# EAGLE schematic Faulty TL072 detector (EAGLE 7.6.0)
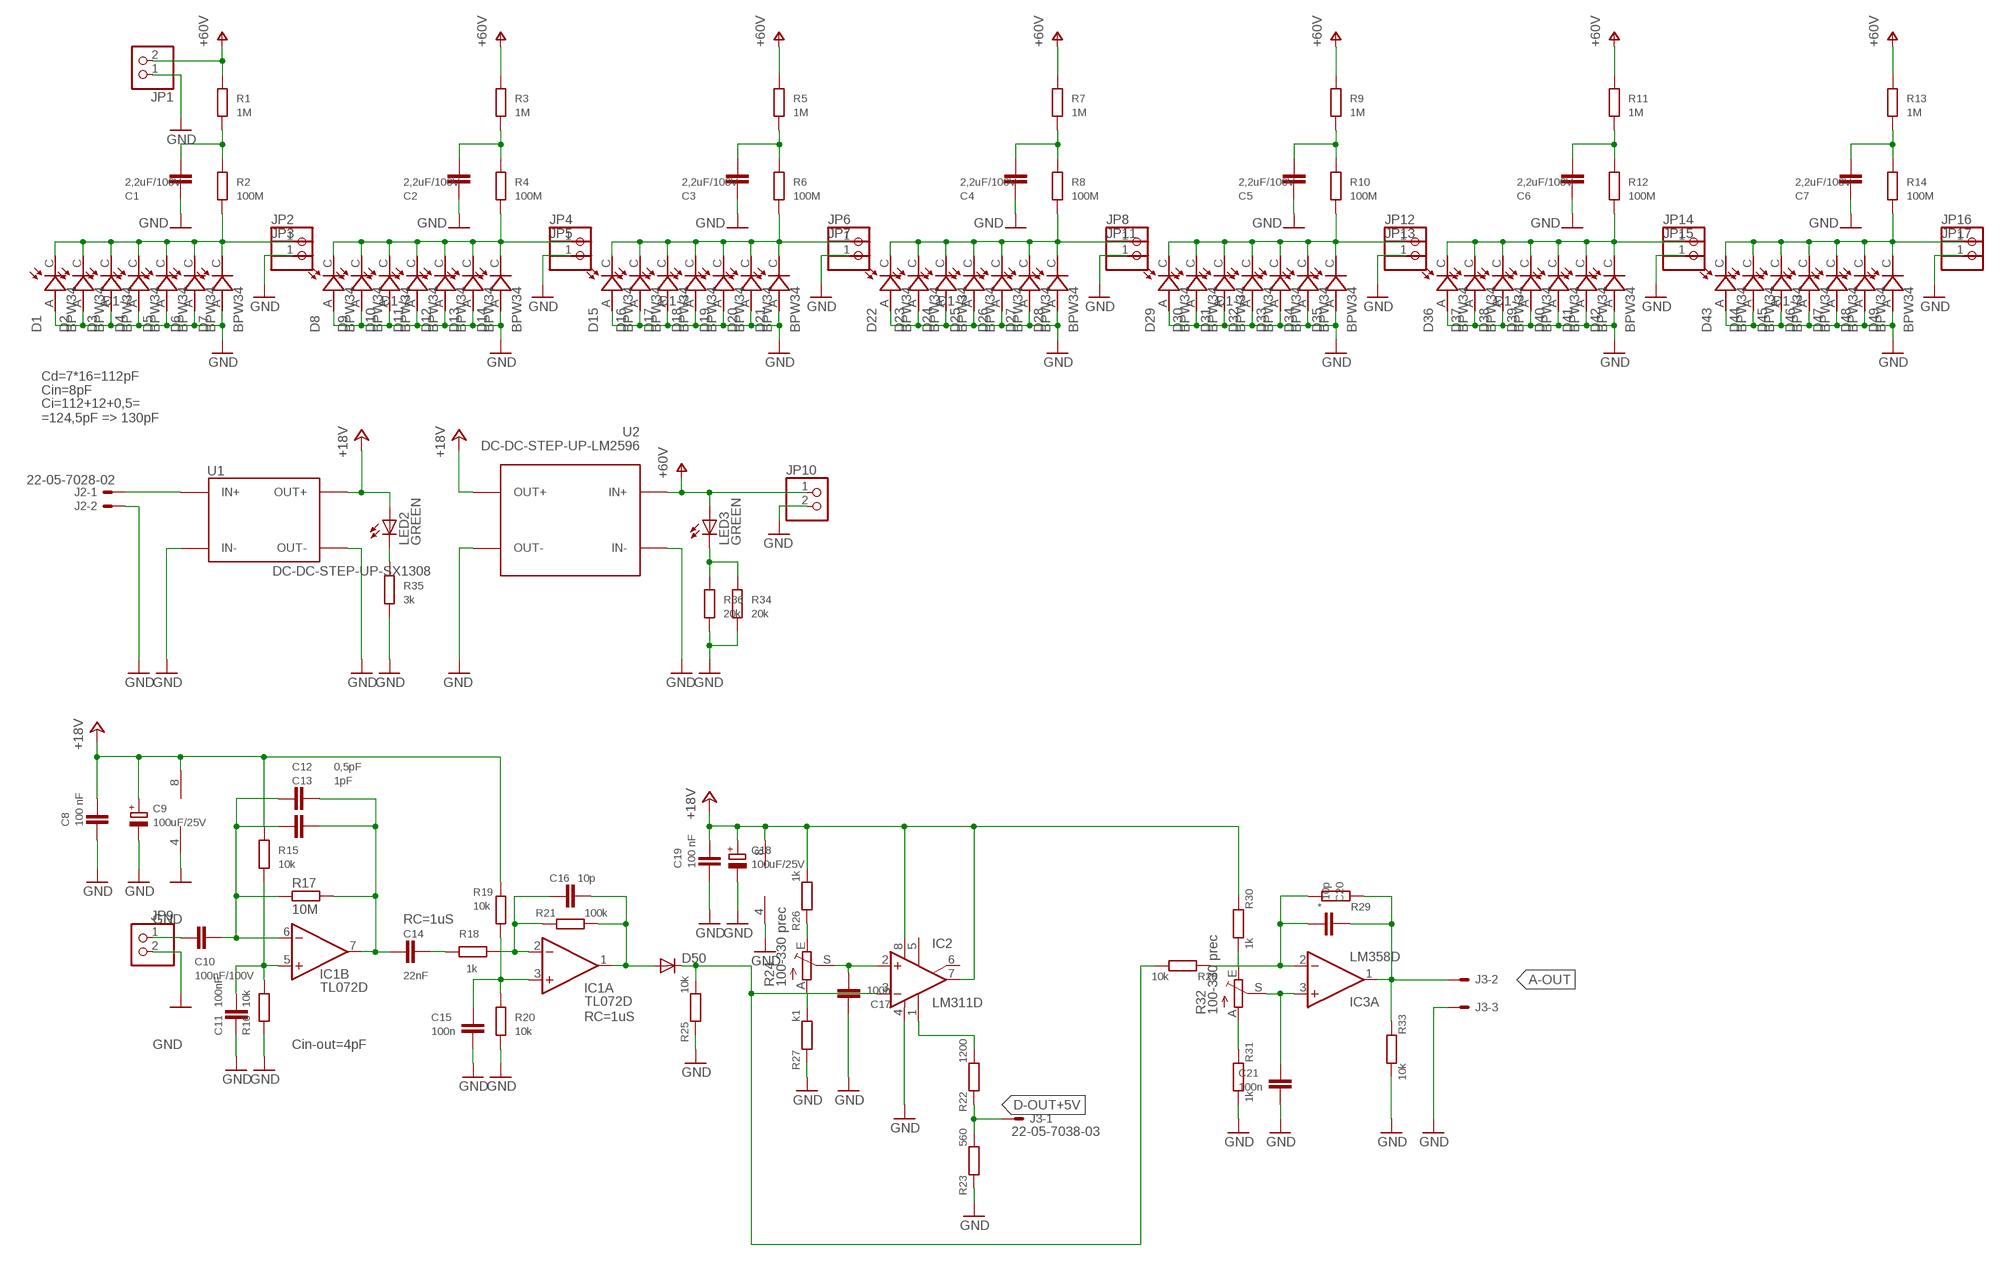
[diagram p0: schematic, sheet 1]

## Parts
C1  2,2uF/100V  C2824  [2824]
C2  2,2uF/100V  C2824  [2824]
C3  2,2uF/100V  C2824  [2824]
C4  2,2uF/100V  C2824  [2824]
C5  2,2uF/100V  C2824  [2824]
C6  2,2uF/100V  C2824  [2824]
C7  2,2uF/100V  C2824  [2824]
C8  100 nF  C-EUC0805  [C0805]
C9  100uF/25V  CPOL-EUSMCD  [SMC_D]
C10  100nF/100V  C-EUC1206  [C1206]
C11  100nF  C-EUC0805  [C0805]
C12  0,5pF  C-EUC0603  [C0603]
C13  1pF  C-EUC0805  [C0805]
C14  22nF  C-EUC0805  [C0805]
C15  100n  C-EUC0805  [C0805]
C16  10p  C-EUC0805  [C0805]
C17  100n  C-EUC0805  [C0805]
C18  100uF/25V  CPOL-EUSMCD  [SMC_D]
C19  100 nF  C-EUC0805  [C0805]
C20  10p  C-EUC0805  [C0805]
C21  100n  C-EUC0805  [C0805]
D1  BPW34  [PHODET_BPW34]
D2  BPW34  [PHODET_BPW34]
D3  BPW34  [PHODET_BPW34]
D4  BPW34  [PHODET_BPW34]
D5  BPW34  [PHODET_BPW34]
D6  BPW34  [PHODET_BPW34]
D7  BPW34  [PHODET_BPW34]
D8  BPW34  [PHODET_BPW34]
D9  BPW34  [PHODET_BPW34]
D10  BPW34  [PHODET_BPW34]
D11  BPW34  [PHODET_BPW34]
D12  BPW34  [PHODET_BPW34]
D13  BPW34  [PHODET_BPW34]
D14  BPW34  [PHODET_BPW34]
D15  BPW34  [PHODET_BPW34]
D16  BPW34  [PHODET_BPW34]
D17  BPW34  [PHODET_BPW34]
D18  BPW34  [PHODET_BPW34]
D19  BPW34  [PHODET_BPW34]
D20  BPW34  [PHODET_BPW34]
D21  BPW34  [PHODET_BPW34]
D22  BPW34  [PHODET_BPW34]
D23  BPW34  [PHODET_BPW34]
D24  BPW34  [PHODET_BPW34]
D25  BPW34  [PHODET_BPW34]
D26  BPW34  [PHODET_BPW34]
D27  BPW34  [PHODET_BPW34]
D28  BPW34  [PHODET_BPW34]
D29  BPW34  [PHODET_BPW34]
D30  BPW34  [PHODET_BPW34]
D31  BPW34  [PHODET_BPW34]
D32  BPW34  [PHODET_BPW34]
D33  BPW34  [PHODET_BPW34]
D34  BPW34  [PHODET_BPW34]
D35  BPW34  [PHODET_BPW34]
D36  BPW34  [PHODET_BPW34]
D37  BPW34  [PHODET_BPW34]
D38  BPW34  [PHODET_BPW34]
D39  BPW34  [PHODET_BPW34]
D40  BPW34  [PHODET_BPW34]
D41  BPW34  [PHODET_BPW34]
D42  BPW34  [PHODET_BPW34]
D43  BPW34  [PHODET_BPW34]
D44  BPW34  [PHODET_BPW34]
D45  BPW34  [PHODET_BPW34]
D46  BPW34  [PHODET_BPW34]
D47  BPW34  [PHODET_BPW34]
D48  BPW34  [PHODET_BPW34]
D49  BPW34  [PHODET_BPW34]
D50  DIODE-SOD323-W  [SOD323-W]
IC1  TL072D  [SO08]
IC2  LM311D  [SO08]
IC3  LM358D  [SO08]
J2  22-05-7028-02  [7395-02]
J3  22-05-7038-03  [7395-03]
JP1  PINHD-1X2  [1X02]
JP2  PINHD-1X1  [1X01]
JP3  PINHD-1X1  [1X01]
JP4  PINHD-1X1  [1X01]
JP5  PINHD-1X1  [1X01]
JP6  PINHD-1X1  [1X01]
JP7  PINHD-1X1  [1X01]
JP8  PINHD-1X1  [1X01]
JP9  PINHD-1X2  [1X02]
JP10  PINHD-1X2  [1X02]
JP11  PINHD-1X1  [1X01]
JP12  PINHD-1X1  [1X01]
JP13  PINHD-1X1  [1X01]
JP14  PINHD-1X1  [1X01]
JP15  PINHD-1X1  [1X01]
JP16  PINHD-1X1  [1X01]
JP17  PINHD-1X1  [1X01]
LED2  GREEN  LEDCHIPLED_1206  [CHIPLED_1206]
LED3  GREEN  LEDCHIPLED_1206  [CHIPLED_1206]
R1  1M  R-EU_M0805  [M0805]
R2  100M  R-EU_R0805  [R0805]
R3  1M  R-EU_M0805  [M0805]
R4  100M  R-EU_R0805  [R0805]
R5  1M  R-EU_M0805  [M0805]
R6  100M  R-EU_R0805  [R0805]
R7  1M  R-EU_M0805  [M0805]
R8  100M  R-EU_R0805  [R0805]
R9  1M  R-EU_M0805  [M0805]
R10  100M  R-EU_R0805  [R0805]
R11  1M  R-EU_M0805  [M0805]
R12  100M  R-EU_R0805  [R0805]
R13  1M  R-EU_M0805  [M0805]
R14  100M  R-EU_R0805  [R0805]
R15  10k  R-EU_R0805  [R0805]
R16  10k  R-EU_R0805  [R0805]
R17  10M  R-EU_R0805  [R0805]
R18  1k  R-EU_R0805  [R0805]
R19  10k  R-EU_R0805  [R0805]
R20  10k  R-EU_R0805  [R0805]
R21  100k  R-EU_R0805  [R0805]
R22  1200  R-EU_R0805  [R0805]
R23  560  R-EU_R0805  [R0805]
R24  100-330 prec  TRIM_EU-SP19L  [SP19L]
R25  10k  R-EU_R0805  [R0805]
R26  1k  R-EU_R0805  [R0805]
R27  k1  R-EU_R0805  [R0805]
R28  10k  R-EU_R0805  [R0805]
R29  *  R-EU_R0805  [R0805]
R30  1k  R-EU_R0805  [R0805]
R31  1k  R-EU_R0805  [R0805]
R32  100-330 prec  TRIM_EU-SP19L  [SP19L]
R33  10k  R-EU_R0805  [R0805]
R34  20k  R-EU_R0805  [R0805]
R35  3k  R-EU_R0805  [R0805]
R36  20k  R-EU_R0805  [R0805]
U1  DC-DC-STEP-UP-SX1308  [DC-DC-STEP-UP-SX1308]
U2  DC-DC-STEP-UP-LM2596  DC-DC-STEP-DOWN-LM2596  [DC-DC-STEP-DOWN-LM2596]

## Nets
+18V: C8.1 C9.+ C18.+ C19.1 IC1.8(P:V+) IC2.7(OUT) IC2.8(V+) IC3.8(P:V+) LED2.A R15.1 R19.1 R26.1 R30.2 U1.OUT+
+24V: U2.OUT+ ; supply symbol labelled +18V
+60: JP1.2 R1.1 R3.1 R5.1 R7.1 R9.1 R11.1 R13.1 ; supply symbol labelled +60V
+60V: JP10.1 LED3.A U2.IN+
A-OUT: C20.2 IC3.1(A:OUT) J3.2 R29.2 R33.2
D-OUT+5V: J3.1 R22.2 R23.1
GND: C1.2 C2.2 C3.2 C4.2 C5.2 C6.2 C7.2 C8.2 C9.- C11.1 C15.1 C17.2 C18.- C19.2 C21.1 D1.A D2.A D3.A D4.A D5.A D6.A D7.A D8.A D9.A D10.A D11.A D12.A D13.A D14.A D15.A D16.A D17.A D18.A D19.A D20.A D21.A D22.A D23.A D24.A D25.A D26.A D27.A D28.A D29.A D30.A D31.A D32.A D33.A D34.A D35.A D36.A D37.A D38.A D39.A D40.A D41.A D42.A D43.A D44.A D45.A D46.A D47.A D48.A D49.A IC1.4(P:V-) IC2.4(V-) IC3.4(P:V-) J2.2 J3.3 JP1.1 JP3.1 JP5.1 JP7.1 JP9.2 JP10.2 JP11.1 JP13.1 JP15.1 JP17.1 R16.2 R20.2 R23.2 R25.2 R27.2 R31.1 R33.1 R34.2 R35.2 R36.2 U1.IN- U1.OUT- U2.IN- U2.OUT-
N$1: C11.2 IC1.5(B:+IN) R15.2 R16.1
N$3: C12.1 C13.1 C14.1 IC1.7(B:OUT) R17.1
N$4: J2.1 U1.IN+
N$5: C1.1 R1.2 R2.1
N$6: C15.2 IC1.3(A:+IN) R19.2 R20.1
N$7: C14.2 R18.2
N$8: C10.2 C12.2 C13.2 IC1.6(B:-IN) R17.2
N$9: C16.2 IC1.2(A:-IN) R18.1 R21.2
N$10: C16.1 D50.A IC1.1(A:OUT) R21.1
N$12: C10.1 JP9.1
N$13: C2.1 R3.2 R4.1
N$14: C3.1 R5.2 R6.1
N$15: C4.1 R7.2 R8.1
N$16: C5.1 R9.2 R10.1
N$17: C6.1 R11.2 R12.1
N$18: C7.1 R13.2 R14.1
N$22: D50.C IC2.3(-IN) R25.1 R28.1
N$23: IC2.1(GND) R22.1
N$24: C20.1 IC3.2(A:-IN) R28.2 R29.1
N$25: C17.1 IC2.2(+IN) R24.S
N$26: R24.E R26.2
N$27: R24.A R27.1
N$29: R30.1 R32.E
N$30: R31.2 R32.A
N$31: C21.2 IC3.3(A:+IN) R32.S
N$32: LED2.C R35.1
N$34: LED3.C R34.1 R36.1
OUT: D1.C D2.C D3.C D4.C D5.C D6.C D7.C JP2.1 R2.2
OUT1: D8.C D9.C D10.C D11.C D12.C D13.C D14.C JP4.1 R4.2
OUT2: D15.C D16.C D17.C D18.C D19.C D20.C D21.C JP6.1 R6.2
OUT3: D22.C D23.C D24.C D25.C D26.C D27.C D28.C JP8.1 R8.2
OUT4: D29.C D30.C D31.C D32.C D33.C D34.C D35.C JP12.1 R10.2
OUT5: D36.C D37.C D38.C D39.C D40.C D41.C D42.C JP14.1 R12.2
OUT6: D43.C D44.C D45.C D46.C D47.C D48.C D49.C JP16.1 R14.2
Unconnected: IC2.5(ON) IC2.6(ON/STR) IC3.5(B:+IN) IC3.6(B:-IN) IC3.7(B:OUT)

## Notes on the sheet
- D1-7 | D1-7 | D1-7 | D1-7 | D1-7 | D1-7 | D1-7
- Cd=7*16=112pF
- Cin=8pF
- Ci=112+12+0,5=
  =124,5pF => 130pF
- RC=1uS
- RC=1uS
- Cin-out=4pF

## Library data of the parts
C1-C7 = capacitor-wima:C: CAPACITOR
C8 C19 = resistor:C-EU: CAPACITOR, European symbol
C9 C18 = rcl:CPOL-EU: POLARIZED CAPACITOR, European symbol
C10-C17 C20 C21 = rcl:C-EU: CAPACITOR, European symbol
D1-D49 = BPW34:BPW34: PIN IR photodiode; DIL; 400-1100nm; 150mW; 60°; λp max:; AVAILABILITY: Good; DESCRIPTION: 950 nm 100 ns %C2%B1 65%C2%B0 Wide Angle Half Sensitivity TO-5 Silicon PIN Photodiode; MF: Vishay; MP: BPW34; PACKAGE: SMD-2 Vishay; PRICE: 0.62 USD
D50 = diode:DIODE-: DIODE
IC1 = linear:TL072: OP AMP
IC2 = linear:LM311: COMPARATOR
IC3 = linear:LM358: OP AMP also LM158; LM258; LM2904 Source: http://cache.national.com/ds/LM/LM158.pdf
J2 = con-molex:22-?-02: CONNECTOR; OC_FARNELL: 9731601; OC_NEWARK: unknown
J3 = con-molex:22-?-03: CONNECTOR wire to board 2.54 mm (.1 inch) pitch header; OC_FARNELL: unknown; OC_NEWARK: unknown
JP1 JP9 JP10 = pinhead:PINHD-1X2: PIN HEADER
JP2-JP8 JP11-JP17 = pinhead:PINHD-1X1: PIN HEADER
LED2 LED3 = led:LED: LED
R1-R23 R25-R31 R33-R36 = rcl:R-EU_: RESISTOR, European symbol
R24 R32 = pot:TRIM_EU-: POTENTIOMETER
U1 = diy-modules:DC-DC-STEP-UP-SX1308
U2 = diy-modules:DC-DC-STEP-DOWN-LM2596: DC/DC Step-Down Regulator based on LM2596-ADJ chip LM2596 datasheet available here: http://www.ti.com/lit/ds/symlink/lm2596.pdf Click here to find device on ebay.com

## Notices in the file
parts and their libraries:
diy-modules: Released under the Creative Commons Attribution 4.0 International License: http://creativecommons.org/licenses/by/4.0
